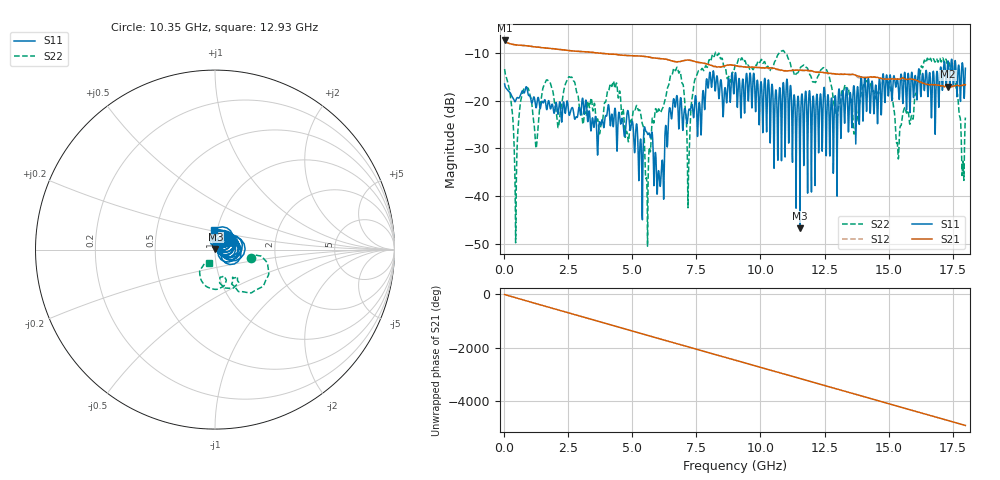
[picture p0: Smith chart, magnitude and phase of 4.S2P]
!Agilent Technologies,E5071C,MY46316741,A.11.02
!Date: Thu Sep 29 15:36:03 2022
!Data & Calibration Information:
!Freq	S11:SOLT2(ON)	S21:SOLT2(ON)	S12:SOLT2(ON)	S22:SOLT2(ON)
!PortZ  Port1:50+j0  Port2:50+j0
!Above PortZ is port z conversion or system Z0 setting when saving the data.
!When reading, reference impedance value at option line is always used.
# Hz S dB R 50
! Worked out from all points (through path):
!   1800 points, 10 MHz to 18 GHz, reference 50 ohm
!   highest |S21| = -7.38 dB at 10 MHz (marker M1); lowest = -17.1 dB at 17.32 GHz (marker M2)
!   group delay of S21, straight-line fit = 757 ps
!   lowest |S11| = -46.8 dB at 11.54 GHz (marker M3), VSWR 1.01, Z = 50.2 + j0.394 ohm
!   |S11| at or under -10 dB: start of sweep to end of sweep
!   |S22| runs from -50.6 to -9.5 dB; largest |S21 - S12| = 0.018
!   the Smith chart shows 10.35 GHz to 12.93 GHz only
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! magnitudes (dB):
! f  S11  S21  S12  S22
! 10 MHz  -16.5  -7.4  -7.4  -13.4
! 440 MHz  -20.1  -8.3  -8.3  -49.9
! 820 MHz  -17.6  -8.5  -8.5  -17.2
! 1.23 GHz  -21.4  -8.7  -8.7  -29.9
! 1.67 GHz  -21.7  -9.0  -9.0  -15.6
! 3.01 GHz  -21.4  -9.7  -9.7  -22.4
! 4.32 GHz  -21.6  -10.3  -10.3  -17.4
! 4.78 GHz  -23.1  -10.5  -10.5  -26.5
! 5.26 GHz  -35.8  -10.6  -10.6  -22.0
! 5.57 GHz  -26.7  -10.8  -10.8  -38.8
! 6.01 GHz  -34.9  -11.1  -11.1  -21.9
! 6.67 GHz  -21.4  -11.8  -11.8  -13.7
! 7.18 GHz  -22.7  -11.5  -11.5  -38.5
! 7.54 GHz  -27.5  -11.9  -12.0  -14.2
! 9.01 GHz  -14.4  -12.7  -12.7  -12.5
! 11.54 GHz  -46.8  -13.6  -13.6  -13.2
! 12.01 GHz  -25.3  -13.8  -13.8  -15.7
! 13.7 GHz  -23.8  -14.6  -14.6  -26.0
! 15.01 GHz  -17.8  -15.5  -15.5  -16.2
! 15.37 GHz  -16.3  -15.5  -15.5  -31.4
! 17.32 GHz  -11.7  -17.1  -17.2  -12.4
! 18 GHz  -13.2  -16.7  -16.8  -23.6
